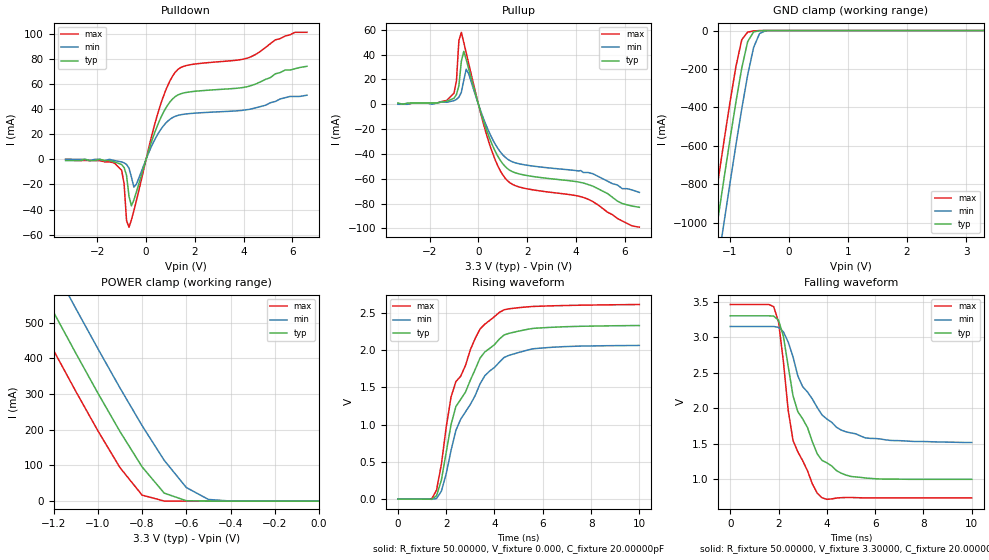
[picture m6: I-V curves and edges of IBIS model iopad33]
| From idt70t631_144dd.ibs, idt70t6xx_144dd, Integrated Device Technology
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|   Model iopad33
[Model]   iopad33
Model_type   I/O
Polarity   Non-Inverting
Enable   Active-Low
Vinl =  0.80000V
Vinh =  2.00000V
Vmeas =  1.50000V
C_comp   4.50000pF   4.50000pF   4.50000pF
[Temperature Range]   25.00000   100.00000   -40.00000
[Voltage Range]   3.30000V   3.10000V   3.50000V
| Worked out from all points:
|   slope of the pulldown table from 0 to 0.495 V, typ, clamps not added: 17.5 ohm
|   slope of the pullup table from 0 to 0.495 V, typ, clamps not added: 16.9 ohm
|   GND clamp passes 1 mA (typ) near -0.50 V on its own axis
|   POWER clamp passes 1 mA (typ) near -0.59 V on its own axis
|   rising waveform, R_fixture 50.00000, V_fixture 0.000, C_fixture 20.00000pF: 20-80 % time 1.45ns typ, 1.54ns min, 1.29ns max; typ from 0 V to 2.33 V
|   falling waveform, R_fixture 50.00000, V_fixture 3.30000, C_fixture 20.00000pF: 20-80 % time 1.2ns typ, 1.52ns min, 857ps max; typ from 3.3 V to 1 V
[Pulldown]
| voltage   I(typ)   I(min)   I(max)
-3.3V     -1mA       0A         0A
-1.5V     -1mA       0A         -2mA
-1V       -4.2mA     -2.1mA     -8.8mA
-900mV    -6.6mA     -2.8mA     -19.7mA
-800mV    -12.8mA    -4.1mA     -48.76mA
-700mV    -29.43mA   -7mA       -53.96mA
-600mV    -37.03mA   -14.17mA   -48.13mA
-500mV    -32.29mA   -22.11mA   -40.89mA
500mV     28.49mA    20.63mA    37.7mA
1.2V      49.93mA    34.24mA    69.32mA
4.1V      57.54mA    39.4mA     80.21mA
6.6V      74mA       51mA       101mA
[Pullup]
| voltage   I(typ)   I(min)   I(max)
-3.3V     1mA        0A         0A
-1.7V     1mA        1mA        1mA
-1V       4.9mA      2.9mA      8.9mA
-900mV    7.8mA      3.9mA      18.89mA
-800mV    14.94mA    5.7mA      51.34mA
-700mV    34.57mA    9.6mA      57.95mA
-600mV    42.62mA    19.25mA    49.81mA
-500mV    36.06mA    28.2mA     41.39mA
400mV     -24.39mA   -20.73mA   -28.72mA
1.1V      -50.2mA    -42.72mA   -59.63mA
4.3V      -63.4mA    -55mA      -75.04mA
6.6V      -83mA      -71mA      -99mA
[GND_clamp]
| voltage   I(typ)   I(min)   I(max)
-3.3V     -5.469A    -5.686A    -5.287A
-1.4V     -1.389A    -1.618A    -1.194A
-1.3V     -1.179A    -1.409A    -984.5mA
-1.2V     -972.3mA   -1.201A    -776.5mA
-1.1V     -767.3mA   -996.6mA   -571.8mA
-900mV    -372.8mA   -596.6mA   -188.1mA
-800mV    -194.3mA   -406.4mA   -47.16mA
-700mV    -57.22mA   -230.7mA   -8.4mA
-600mV    -7.393mA   -88.33mA   -2.169mA
-500mV    -1.009mA   -16.09mA   -229.2uA
-400mV    -92.71uA   -1.476mA   -9.663uA
3.3V      525.2pA    638.3nA    1.93pA
[POWER_clamp]
| voltage   I(typ)   I(min)   I(max)
-3.3V     3.039A     3.158A     2.94A
-1.4V     762.6mA    887.5mA    656.3mA
-1.3V     645.8mA    771mA      539.1mA
-1.2V     529.9mA    655.3mA    422.9mA
-1.1V     415.5mA    540.8mA    308.5mA
-1V       303.3mA    427.9mA    197.7mA
-900mV    195.4mA    317.6mA    94.25mA
-800mV    96.26mA    211.9mA    16.94mA
-700mV    22.53mA    114.6mA    304.8uA
-600mV    1.137mA    38.18mA    3.7uA
-500mV    27.9uA     4.729mA    76.79nA
0V        525.2pA    48.85nA    2.01pA
[Ramp]
| variable   typ   min   max
dV/dt_r   1.40040/0.58697n   1.23900/0.67661n   1.57020/0.47442n
dV/dt_f   1.38174/0.37674n   1.05360/0.46010n   1.62528/0.29291n
R_load = 50.00000
[Rising Waveform]
R_fixture = 50.00000
V_fixture = 0.000
C_fixture = 20.00000pF
R_dut = 0.11800
L_dut = 6.90000nH
C_dut = 1.23000pF
| time   V(typ)   V(min)   V(max)
0s        0V         0V         0V
1.4ns     -2.401mV   -3.579mV   3.115mV
1.6ns     45.13mV    7.529mV    120.3mV
1.8ns     254.4mV    106.1mV    465.5mV
2.2ns     998.9mV    652.6mV    1.369V
2.4ns     1.241V     921.1mV    1.575V
3.4ns     1.891V     1.545V     2.28V
4.2ns     2.146V     1.835V     2.504V
5.6ns     2.289V     2.016V     2.584V
10ns      2.328V     2.061V     2.61V
[Falling Waveform]
R_fixture = 50.00000
V_fixture = 3.30000
C_fixture = 20.00000pF
R_dut = 0.11800
L_dut = 6.90000nH
C_dut = 1.23000pF
| time   V(typ)   V(min)   V(max)
0s        3.3V       3.15V      3.459V
1.8ns     3.295V     3.15V      3.429V
2ns       3.237V     3.138V     3.215V
2.2ns     3.014V     3.075V     2.658V
2.4ns     2.589V     2.93V      1.97V
2.6ns     2.174V     2.722V     1.546V
3ns       1.85V      2.303V     1.261V
3.8ns     1.266V     1.906V     739.8mV
5.6ns     1.018V     1.581V     738.5mV
10ns      1V         1.518V     738.8mV
